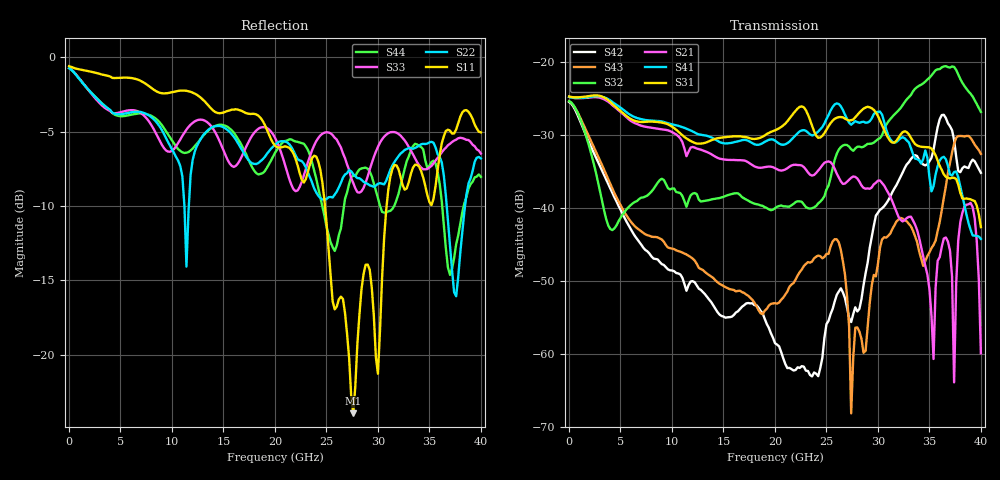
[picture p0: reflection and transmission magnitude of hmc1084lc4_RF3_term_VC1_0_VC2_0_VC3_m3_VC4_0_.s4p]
!Agilent Technologies,N5224A,MY51441122,A.09.40.06
!Agilent N5224A: A.09.40.06
!Date: Thursday, June 19, 2014 00:51:01
!Correction: S11(Full 4 Port(1,2,3,4))
!S12(Full 4 Port(1,2,3,4))
!S13(Full 4 Port(1,2,3,4))
!S14(Full 4 Port(1,2,3,4))
!S21(Full 4 Port(1,2,3,4))
!S22(Full 4 Port(1,2,3,4))
!S23(Full 4 Port(1,2,3,4))
!S24(Full 4 Port(1,2,3,4))
!S31(Full 4 Port(1,2,3,4))
!S32(Full 4 Port(1,2,3,4))
!S33(Full 4 Port(1,2,3,4))
!S34(Full 4 Port(1,2,3,4))
!S41(Full 4 Port(1,2,3,4))
!S42(Full 4 Port(1,2,3,4))
!S43(Full 4 Port(1,2,3,4))
!S44(Full 4 Port(1,2,3,4))
!S4P File: Measurements: <S11,S12,S13,S14>,
!<S21,S22,S23,S24>,
!<S31,S32,S33,S34>,
!<S41,S42,S43,S44>:
# Hz S  dB  R 50
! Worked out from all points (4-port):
!   201 points, 10 MHz to 40 GHz, reference 50 ohm
!   strongest paths, dB at 10 MHz, 10.01 GHz, 20 GHz, 30 GHz, 40 GHz:
!     S31: -24.7, -28.9, -29.4, -27.4, -42.6
!     S41: -24.8, -28.5, -30.8, -26.8, -44.2
!     S21: -24.8, -29.6, -34.6, -36.3, -59.9
!     S32: -25.4, -37.3, -40.0, -30.6, -26.8
!     S43: -25.4, -45.6, -53.0, -47.6, -32.6
!     S42: -25.5, -48.6, -58.5, -40.7, -35.2
!   lowest |S11| = -23.9 dB at 27.6 GHz (marker M1), VSWR 1.14, Z = 55.8 + j3.48 ohm
!   |S11| at or under -10 dB: 24.86 GHz to 30.84 GHz (5.985 GHz wide, 21.5 % of centre)
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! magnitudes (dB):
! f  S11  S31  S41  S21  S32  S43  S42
! 10 MHz  -0.6  -24.7  -24.8  -24.8  -25.4  -25.4  -25.5
! 27.6 GHz  -23.9  -27.9  -28.3  -35.7  -32.2  -60.5  -54.5
! 35.4 GHz  -9.5  -32.3  -37.0  -60.7  -21.5  -45.1  -32.0
! 36.8 GHz  -4.9  -35.9  -34.2  -44.6  -20.7  -35.2  -28.4
! 37.4 GHz  -5.1  -35.9  -35.1  -63.9  -20.7  -31.2  -30.7
! 39.2 GHz  -4.1  -38.9  -43.8  -39.9  -24.7  -30.8  -33.4
! 40 GHz  -5.1  -42.6  -44.2  -59.9  -26.8  -32.6  -35.2
